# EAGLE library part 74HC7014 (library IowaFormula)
Hex BUFFER, non-inverting Google Drive Datasheet
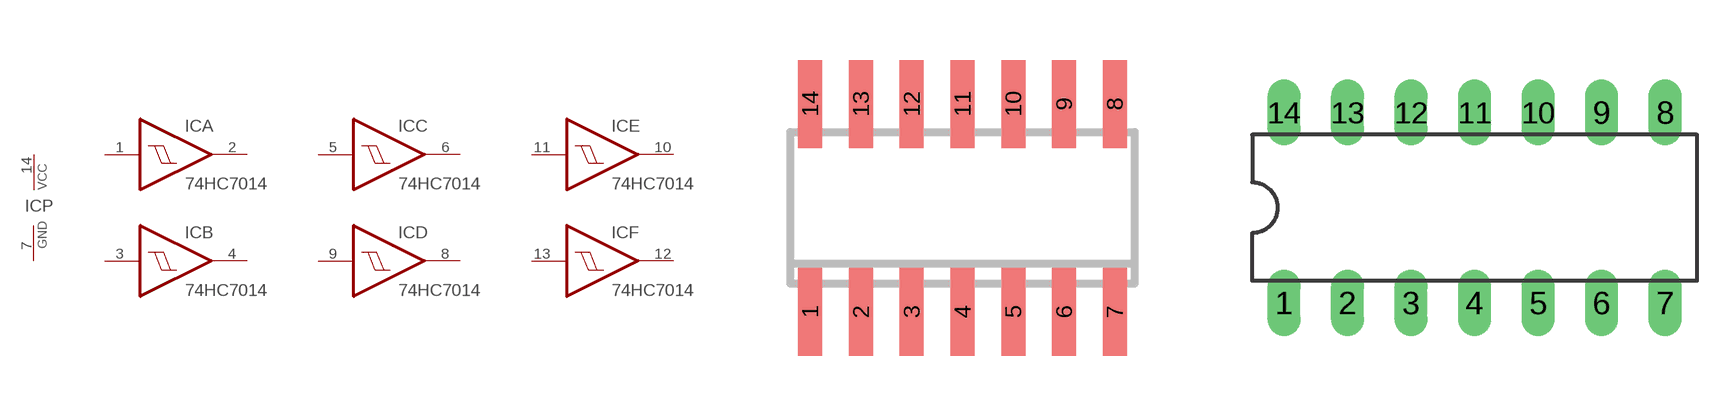
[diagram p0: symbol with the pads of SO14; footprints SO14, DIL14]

Designator prefix IC; gates P=PWR A=7417 B=7417 C=7417 D=7417 E=7417 F=7417

## 74HC7014  [SO14]
1  A:I  in
2  A:O  out
3  B:I  in
4  B:O  out
5  C:I  in
6  C:O  out
7  P:GND  pwr
8  D:O  out
9  D:I  in
10  E:O  out
11  E:I  in
12  F:O  out
13  F:I  in
14  P:VCC  pwr

## 74HC7014DIL14  [DIL14]
Pads as for SO14

## Footprint SO14 (pad centres in mm)
Small Outline Package 14
smd 0.6 x 2.2: 1 -3.81,-2.6; 2 -2.54,-2.6; 3 -1.27,-2.6; 4 0,-2.6; 5 1.27,-2.6; 6 2.54,-2.6; 7 3.81,-2.6; 8 3.81,2.6; 9 2.54,2.6; 10 1.27,2.6; 11 0,2.6; 12 -1.27,2.6; 13 -2.54,2.6; 14 -3.81,2.6

## Footprint DIL14 (pad centres in mm)
Dual In Line Package
drill 0.813 long: 1 -7.62,-3.81; 2 -5.08,-3.81; 3 -2.54,-3.81; 4 0,-3.81; 5 2.54,-3.81; 6 5.08,-3.81; 7 7.62,-3.81; 8 7.62,3.81; 9 5.08,3.81; 10 2.54,3.81; 11 0,3.81; 12 -2.54,3.81; 13 -5.08,3.81; 14 -7.62,3.81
